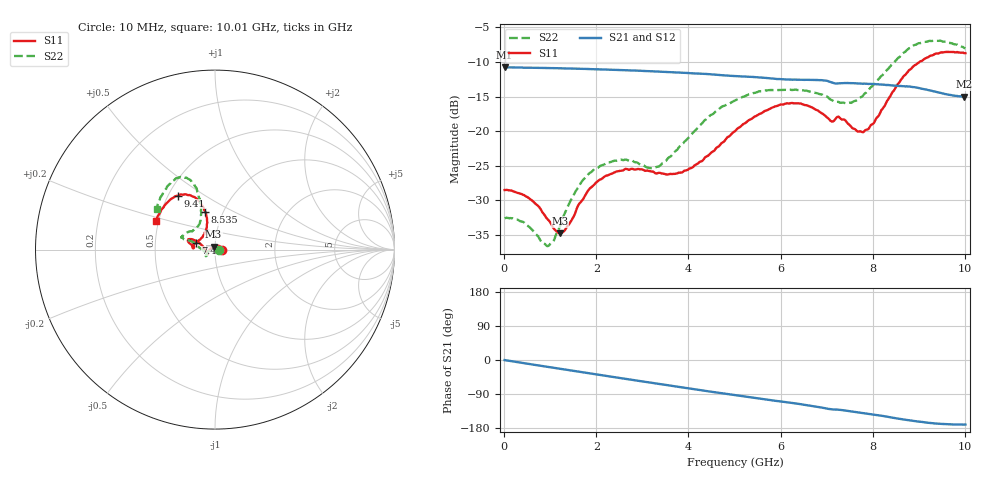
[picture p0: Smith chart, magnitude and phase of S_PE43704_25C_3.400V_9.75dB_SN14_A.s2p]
! Device ID: PE43704
! Dir: z:\PE43704\PE43704_Char_1_20130516\PE43704\AMB\3p400V\9p75dB
! Serial: 14
! Insertion: A
! Impedance: 50 ohm
! Temp: Amb
! VDD: 3.400V
! Attenuation Step: 9.75dB
! IDD: 1.140414e-01mA
#  Hz  S  RI  R  50
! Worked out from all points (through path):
!   401 points, 10 MHz to 10.01 GHz, reference 50 ohm
!   highest |S21| = -10.77 dB at 10 MHz (marker M1); lowest = -15.0 dB at 9.985 GHz (marker M2)
!   group delay of S21, straight-line fit = 49 ps
!   lowest |S11| = -34.8 dB at 1.21 GHz (marker M3), VSWR 1.04, Z = 49.2 + j1.62 ohm
!   |S11| at or under -10 dB: start of sweep to 9.014 GHz
!   |S22| runs from -36.6 to -6.9 dB; largest |S21 - S12| = 0.0023
!   S11 on the Smith chart (normalised r, x): 10 MHz: 1.08, +0.00; 7.46 GHz: 0.81, +0.06; 8.535 GHz: 0.82, +0.36; 9.41 GHz: 0.56, +0.39; 10.01 GHz: 0.48, +0.18
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1e7  0.0375 0.00026  0.2895 -0.00112  0.2897 -0.001  0.0234 0.000271
5.1e8  0.0277 0.0184  0.2831 -0.0493  0.283 -0.0492  0.0145 0.0147
9.35e8  0.00767 0.0219  0.2718 -0.0879  0.2718 -0.0877  -0.00437 0.0141
1.21e9  -0.00784 0.0165  0.2617 -0.1119  0.2616 -0.1118  -0.0195 0.0061
1.385e9  -0.0178 0.0106  0.2539 -0.1263  0.254 -0.1263  -0.0286 -0.001
1.685e9  -0.0313 -0.0014  0.2389 -0.1499  0.2389 -0.1498  -0.0404 -0.0154
2.01e9  -0.0406 -0.0136  0.22 -0.1729  0.2201 -0.1728  -0.0457 -0.0284
2.41e9  -0.0443 -0.0246  0.1939 -0.198  0.194 -0.1978  -0.0495 -0.0359
3.36e9  -0.0436 -0.0243  0.1217 -0.2401  0.122 -0.24  -0.0532 -0.016
4.035e9  -0.0538 -0.00105  0.0658 -0.2538  0.0663 -0.2538  -0.0906 0.0145
5.01e9  -0.0919 0.0391  -0.0117 -0.2496  -0.0114 -0.25  -0.1584 0.0516
5.96e9  -0.1418 0.0594  -0.0765 -0.2254  -0.0758 -0.2255  -0.1862 0.0676
6.685e9  -0.1437 0.0364  -0.1219 -0.2004  -0.1219 -0.2002  -0.173 0.0832
7.085e9  -0.1173 0.0174  -0.1445 -0.1742  -0.1452 -0.1746  -0.1349 0.1021
7.46e9  -0.1062 0.0392  -0.156 -0.1589  -0.1558 -0.159  -0.1011 0.1248
7.86e9  -0.0655 0.0788  -0.1714 -0.1373  -0.1716 -0.138  -0.0794 0.1731
8.36e9  -0.0446 0.1689  -0.1873 -0.1053  -0.1864 -0.1062  -0.084 0.2759
8.535e9  -0.055 0.2101  -0.1917 -0.0922  -0.1902 -0.0935  -0.0979 0.3196
8.935e9  -0.1031 0.2839  -0.1964 -0.0652  -0.1955 -0.063  -0.1493 0.394
9.41e9  -0.2049 0.3003  -0.1868 -0.0396  -0.1863 -0.0388  -0.229 0.3864
9.985e9  -0.3239 0.1699  -0.1749 -0.0298  -0.1758 -0.0297  -0.3212 0.2366
1.001e10  -0.3295 0.1596  -0.1752 -0.0301  -0.1768 -0.0305  -0.3246 0.2286
